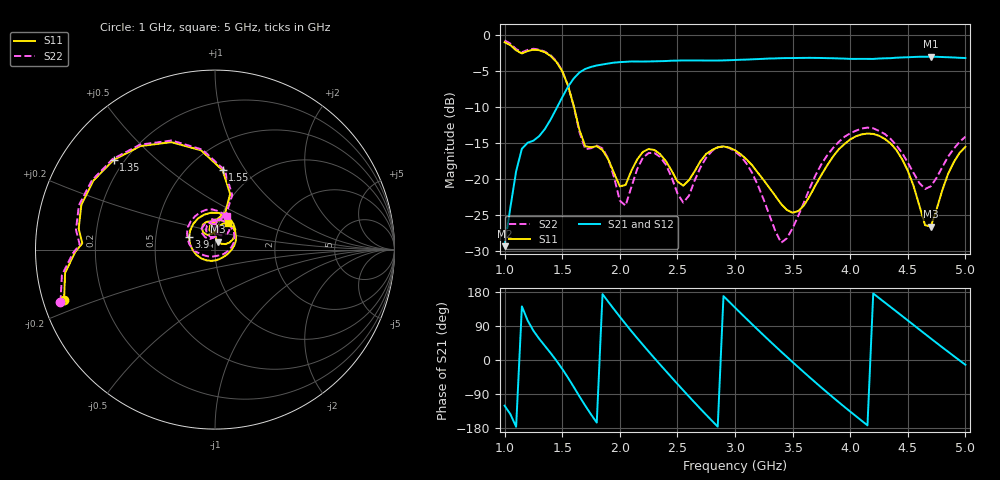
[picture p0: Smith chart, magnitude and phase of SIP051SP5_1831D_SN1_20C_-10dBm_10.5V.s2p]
# GHz  S  dB  R  50
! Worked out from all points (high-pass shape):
!   81 points, 1 GHz to 5 GHz, reference 50 ohm
!   highest |S21| = -3.07 dB at 4.7 GHz (marker M1); lowest = -29.3 dB at 1 GHz (marker M2)
!   |S21| within 3 dB of the highest: 1.6 GHz to end of sweep
!   lowest |S11| = -26.6 dB at 4.7 GHz (marker M3), VSWR 1.10, Z = 51.6 + j4.51 ohm
!   |S11| at or under -10 dB: 1.602 GHz to end of sweep
!   |S22| runs from -28.8 to -0.8 dB; largest |S21 - S12| = 0.0025
!   S11 on the Smith chart (normalised r, x): 1 GHz: 0.06, -0.16; 1.35 GHz: 0.16, +0.37; 1.55 GHz: 0.72, +0.80; 3.9 GHz: 0.74, +0.11; 5 GHz: 1.10, +0.34
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1  -1.05 -161.7  -29.27 -120.5  -29.17 -120.0  -0.82 -161.1
1.15  -2.61 177.3  -15.80 141.5  -15.81 141.2  -2.45 177.9
1.35  -2.45 138.5  -13.06 37.0  -13.05 36.9  -2.37 138.5
1.55  -7.04 84.5  -7.23 -46.5  -7.23 -46.5  -7.03 83.0
1.7  -15.45 85.9  -4.76 -120.5  -4.77 -120.4  -15.85 86.7
1.85  -15.99 91.4  -4.14 173.9  -4.14 173.8  -15.76 88.9
2.05  -20.80 117.1  -3.77 95.1  -3.78 95.1  -23.67 114.8
2.2  -16.24 116.0  -3.74 40.1  -3.73 40.0  -17.04 121.8
2.35  -16.55 91.1  -3.69 -12.1  -3.69 -12.1  -16.94 93.1
2.6  -20.16 103.0  -3.58 -96.2  -3.58 -96.2  -22.30 110.2
2.8  -15.98 87.8  -3.60 -160.4  -3.60 -160.4  -16.11 99.3
3  -16.00 50.2  -3.52 138.4  -3.51 138.4  -16.18 55.4
3.2  -19.15 12.8  -3.39 79.4  -3.40 79.3  -20.90 7.0
3.4  -23.43 -29.1  -3.27 22.1  -3.27 22.2  -28.80 -72.0
3.55  -24.41 -85.8  -3.24 -19.2  -3.23 -19.2  -25.05 -138.8
3.7  -20.82 -147.2  -3.23 -59.5  -3.23 -59.4  -19.43 -173.6
3.9  -15.89 154.3  -3.31 -111.2  -3.32 -111.2  -14.87 149.5
4.15  -13.70 95.9  -3.37 -172.4  -3.37 -172.4  -12.87 102.8
4.35  -15.05 54.5  -3.27 140.0  -3.27 140.0  -14.43 69.4
4.55  -20.94 25.8  -3.11 92.5  -3.10 92.5  -19.14 52.9
4.7  -26.55 67.9  -3.07 56.8  -3.06 56.8  -20.99 84.1
5  -15.53 64.2  -3.25 -12.5  -3.25 -12.4  -14.13 69.8
